PROGRAM MAIN
VAR
	bError						: BOOL;					// True if modules have errors
		(***** Axis variable *****)
	lrAxisVelo					: LREAL;
		
		(***** Variables of state machine *****)
	bStarted					: BOOL;					// True if state machine is in state EXECUTE
	bStopped					: BOOL;					// True if state machine is in state STOPPED
	bReset						AT %Q*: BOOL;			// True if state machine is in state RESETTING
	bAborted					: BOOL;					// True if state machine is in state ABORTED
	bIdle						: BOOL;					// True if state machine is in state IDLE
	bAuto						: BOOL;					// True if state machine is in mode AUTOMATIC
	bSemi						: BOOL;					// True if state machine is in mode SEMIAUTOMATIC
	bManual						: BOOL;					// True if state machine is in mode MANUAL
	bMaintenance				: BOOL;					// True if state machine is in mode MAINTENANCE
	bStartButtonOff				: BOOL;					// To turn off start button

(* ========================== Function block instances =============================== *)

		(**** Machine elements *****)
	fbSeparateModule			: FB_SeparatingModule;			// Separating module
	fbMetalSorting				: FB_SortingModule;				// Module that sorts metal boxes
	fbPlasticSorting			: FB_SortingModule;				// Module that sorts plastic boxes
	fbComprAir					: FB_SignalHandlingIntern;		// Compressed air
	fbPowerSupply				: FB_SignalHandlingIntern;		// Power supply
	fbVisu						: FB_Visu;						// Visualization

		(***** Buttons *****)
	fbButtonStart				: FB_SignalHandlingIntern;		// Button to start the machine
	fbButtonStop				: FB_SignalHandlingIntern;		// Button to stop the machine
	fbButtonReset				: FB_SignalHandlingIntern;		// Button to reset the machine
	fbButtonAbort				: FB_SignalHandlingIntern;		// Button to abort the machine
	fbButtonAuto				: FB_SignalHandlingIntern;		// Button to change machine mode to AUTOMATIC
	fbButtonSemi				: FB_SignalHandlingIntern;		// Button to change machine mode to SEMI-AUTOMATIC
	fbButtonManual				: FB_SignalHandlingIntern;		// Button to change machine mode to MANUAL
	fbButtonMaintenance			: FB_SignalHandlingIntern;		// Button to change machine mode to MAINTENANCE
	fbButtonPower				: FB_SignalHandlingIntern;		// Button to control power supply
	fbButtonComprAir			: FB_SignalHandlingIntern;		// Button to control compressed air

(* ========================== COMMON VARIABLES =============================== *)	

		(***** State machine *****)
	fbStateMachineAuto			: PS_PackML_StateMachine_Auto;			// State machine for mode AUTOMATIC
	fbStateMachineSemiAuto		: PS_PackML_StateMachine_SemiAuto;		// State machine for mode SEMI-AUTOMATIC
	fbStateMachineManual		: PS_PackML_StateMachine_Manual;		// State machine for mode MANUAL
	fbStateMachineMaintenance	: PS_PackML_StateMachine_Maintenance;	// State machine for mode MAINTENANCE
	
	ePMLUnitMode				: E_PMLUnitMode := ePMLUnitMode_IDLE;	// Current mode
	ePMLUnitModeRequested		: E_PMLUnitMode;						// Requested mode
	fbUnitModeManager			: PS_UnitModeManager;					// Mode manager
	ePMLState					: E_PMLState := ePMLState_IDLE;			// Current state
	ePMLStateRequested			: E_PMLState;							// Requested state
	
		(* Common variables *)
	bManualAxisEnable			: BOOL;							// True if it is allowed to move manually axis
	fbTriggerStart				: R_TRIG;						// To diagnose rising edge of start button
	fbTriggerSeparated			: R_TRIG;						// To diagnose rising edge of separated box
	fbTriggerSelectedM			: R_TRIG;						// To diagnose rising edge of selected metal box
	fbTriggerSelectedP			: R_TRIG;						// To diagnose rising edge of selected plastic box
	nBoxesOnTheWay				: INT;							// Number of boxes being moved
	aClampTemps					: ARRAY[1..100] OF LREAL;		// Temperature of clamp cylinder
	aBarrierTemps				: ARRAY[1..100] OF LREAL;		// Temperature of barrier cylinder
	aMetalTemps					: ARRAY[1..100] OF LREAL;		// Temperature of metal cylinder
	aPlasticTemps				: ARRAY[1..100] OF LREAL;		// Temperature of plastic cylinder
	bStartingStart				: BOOL;							// True if state machine is in state STARTING
	bResetStart					: BOOL;							// True if state machine is in state RESETTING
	bHaltStart					: BOOL;							// True if state machine is in state STOPPING
	nHaltTriesSeperate			: INT;
	nHaltTriesMetal				: INT;
	nHaltTriesPlastic			: INT;
END_VAR

// =========================================================
	// Getting errors of modules
	
bError := fbSeparateModule.fbAxis.iErrorID <> 0
			OR fbMetalSorting.fbAxis.iErrorID <> 0
			OR fbPlasticSorting.fbAxis.iErrorID <> 0
			OR fbSeparateModule.bClampError OR fbSeparateModule.bBarrierError
			OR fbMetalSorting.bCylError OR fbPlasticSorting.bCylError;
	
// =========================================================
	// Setting velocities of axes

IF ePMLUnitMode = ePMLUnitMode_AUTOMATIC OR ePMLUnitMode = ePMLUnitMode_SEMIAUTOMATIC THEN
	lrAxisVelo := 100;
ELSE
	lrAxisVelo := 50;
END_IF

// =========================================================
	// Noticing separated and selected boxes
	
fbTriggerSeparated( CLK := fbSeparateModule.bSeparated );
fbTriggerSelectedM( CLK := fbMetalSorting.bSelected );
fbTriggerSelectedP( CLK := fbPlasticSorting.bSelected );
						
// =========================================================
	// Getting cylinder temperatures of modules
	
aBarrierTemps 	:= fbSeparateModule.aBarrierTemps;
aClampTemps 	:= fbSeparateModule.aClampTemps;
aMetalTemps 	:= fbMetalSorting.aTemps;
aPlasticTemps 	:= fbPlasticSorting.aTemps;

// =========================================================
	// Cylinder options of modules
	
fbSeparateModule.M_CylinderOptions();
fbMetalSorting.M_CylinderOptions();
fbPlasticSorting.M_CylinderOptions();

// =========================================================
	// Mode and state requests
A_Requests();

	// Enable for power supply, compressed air control and buttons
A_Enable();

	// Input variables of separating and sorting modules
A_ModuleInputs();

	// Output variables
A_SetOutput();

	// State machine
A_StateMachine();

	// Visualization
A_Visu();

// =========================================================

ACTION A_Semiautomatic:
// =========================================================

CASE ePMLState OF
	
// =========================================================
	// Turning axis reset off, passing it to axis instances
	ePMLState_IDLE:		

				IF bResetStart THEN
					bResetStart 			:= FALSE;
					
					fbSeparateModule.bReset	:= FALSE;
					fbSeparateModule.M_Reset();
					
					fbMetalSorting.bReset 	:= FALSE;
					fbMetalSorting.M_Reset();
					
					fbPlasticSorting.bReset	:= FALSE;
					fbPlasticSorting.M_Reset();
					
					fbStateMachineSemiAuto.StateComplete := FALSE;
				END_IF
	
// =========================================================
	// Resetting variables for executing automatic mode, checking status of axes
	ePMLState_STARTING:	

				IF NOT bStartingStart THEN
					bStartingStart 				:= TRUE;
					
					fbSeparateModule.bStarting	:= TRUE;
					fbSeparateModule.M_Starting();
					
					fbMetalSorting.bStarting 	:= TRUE;
					fbMetalSorting.M_Starting();
					
					fbPlasticSorting.bStarting	:= TRUE;
					fbPlasticSorting.M_Starting();
				END_IF

				IF NOT fbSeparateModule.bStartingDone THEN
					fbSeparateModule.M_Starting();
				END_IF
				
				IF NOT fbMetalSorting.bStartingDone THEN
					fbMetalSorting.M_Starting();
				END_IF
				
				IF NOT fbPlasticSorting.bStartingDone THEN
					fbPlasticSorting.M_Starting();
				END_IF

				IF fbSeparateModule.bStartingDone AND fbMetalSorting.bStartingDone
				AND fbPlasticSorting.bStartingDone THEN
					fbStateMachineSemiAuto.StateComplete := TRUE;
				END_IF

// =========================================================
	// Executing semi-automatic mode
	ePMLState_EXECUTE:	

				IF bStartingStart THEN
					bStartingStart 				:= FALSE;
					
					fbSeparateModule.bStarting 	:= FALSE;
					fbSeparateModule.M_Starting();
					
					fbMetalSorting.bStarting 	:= FALSE;
					fbMetalSorting.M_Starting();
					
					fbPlasticSorting.bStarting 	:= FALSE;
					fbPlasticSorting.M_Starting();
					
					fbStateMachineSemiAuto.StateComplete := FALSE;
				END_IF
				
				fbSeparateModule.M_Semiautomatic();
				fbMetalSorting.M_Semiautomatic();
				fbPlasticSorting.M_Semiautomatic();
				
				IF fbTriggerSeparated.Q THEN
					nBoxesOnTheWay := nBoxesOnTheWay + 1;
				END_IF
				
				IF fbTriggerSelectedM.Q THEN
					nBoxesOnTheWay := nBoxesOnTheWay - 1;
				END_IF
				
				IF fbTriggerSelectedP.Q THEN
					nBoxesOnTheWay := nBoxesOnTheWay - 1;
				END_IF
						
// =========================================================
	// Stopping axes
	ePMLState_ABORTING:	

				IF NOT bHaltStart THEN
					bHaltStart 				:= TRUE;
					
					fbSeparateModule.bHalt 	:= TRUE;
					fbSeparateModule.M_Stop();
					
					fbMetalSorting.bHalt 	:= TRUE;
					fbMetalSorting.M_Stop();
					
					fbPlasticSorting.bHalt 	:= TRUE;
					fbPlasticSorting.M_Stop();						
				END_IF

				IF NOT fbSeparateModule.bHaltDone THEN
					fbSeparateModule.M_Stop();
				END_IF
				
				IF NOT fbMetalSorting.bHaltDone THEN
					fbMetalSorting.M_Stop();
				END_IF
				
				IF NOT fbPlasticSorting.bHaltDone THEN
					fbPlasticSorting.M_Stop();
				END_IF

				IF fbSeparateModule.bHaltDone AND fbMetalSorting.bHaltDone
				AND fbPlasticSorting.bHaltDone THEN
					fbStateMachineSemiAuto.StateComplete := TRUE;
				END_IF
	
// =========================================================
	// Turning off axis stop, passing it to axis instances
	ePMLState_ABORTED:	

				IF fbStateMachineSemiAuto.StateComplete THEN
					fbStateMachineSemiAuto.StateComplete := FALSE;
				END_IF
				
				IF bHaltStart THEN
					bHaltStart 				:= FALSE;
					
					fbSeparateModule.bHalt 	:= FALSE;
					fbSeparateModule.M_Stop();
					
					fbMetalSorting.bHalt 	:= FALSE;
					fbMetalSorting.M_Stop();
					
					fbPlasticSorting.bHalt 	:= FALSE;
					fbPlasticSorting.M_Stop();
				END_IF
	
// =========================================================
	ePMLState_CLEARING:	

				fbStateMachineSemiAuto.StateComplete := TRUE;
	
// =========================================================
	// Selecting boxes on conveyor belt to destination, then stopping axes
	ePMLState_STOPPING:	

				IF fbTriggerSeparated.Q THEN
					nBoxesOnTheWay := nBoxesOnTheWay + 1;
				END_IF
				
				IF fbTriggerSelectedM.Q THEN
					nBoxesOnTheWay := nBoxesOnTheWay - 1;
				END_IF
				
				IF fbTriggerSelectedP.Q THEN
					nBoxesOnTheWay := nBoxesOnTheWay - 1;
				END_IF
				
				IF nBoxesOnTheWay = 0 AND NOT bHaltStart THEN
					bHaltStart				:= TRUE;
					
					fbSeparateModule.bHalt 	:= TRUE;
					fbSeparateModule.M_Stop();
					
					fbMetalSorting.bHalt 	:= TRUE;
					fbMetalSorting.M_Stop();
					
					fbPlasticSorting.bHalt 	:= TRUE;
					fbPlasticSorting.M_Stop();						
				END_IF
				
				IF NOT fbSeparateModule.bHaltDone OR nBoxesOnTheWay <> 0 THEN
					fbSeparateModule.M_Automatic();
				END_IF
				
				IF NOT fbMetalSorting.bHaltDone OR nBoxesOnTheWay <> 0 THEN
					fbMetalSorting.M_Automatic();
				END_IF
				
				IF NOT fbPlasticSorting.bHaltDone OR nBoxesOnTheWay <> 0 THEN
					fbPlasticSorting.M_Automatic();
				END_IF

				IF fbSeparateModule.bHaltDone AND fbMetalSorting.bHaltDone
				AND fbPlasticSorting.bHaltDone AND nBoxesOnTheWay = 0 THEN
					fbStateMachineSemiAuto.StateComplete := TRUE;
				END_IF
					
// =========================================================
	// Turning off axis stop, passing it to axis instances
	ePMLState_STOPPED:	

				IF fbStateMachineSemiAuto.StateComplete THEN
					fbStateMachineSemiAuto.StateComplete := FALSE;
				END_IF
				
				IF bHaltStart THEN
					bHaltStart 				:= FALSE;
					
					fbSeparateModule.bHalt 	:= FALSE;
					fbSeparateModule.M_Stop();
					
					fbMetalSorting.bHalt 	:= FALSE;
					fbMetalSorting.M_Stop();
					
					fbPlasticSorting.bHalt 	:= FALSE;
					fbPlasticSorting.M_Stop();
				END_IF

// =========================================================
	// Resetting cylinders and axes
	ePMLState_RESETTING:	

				IF NOT bResetStart THEN
					bResetStart				:= TRUE;
					
					fbSeparateModule.bReset	:= TRUE;
					fbSeparateModule.M_Reset();
					
					fbMetalSorting.bReset 	:= TRUE;
					fbMetalSorting.M_Reset();
					
					fbPlasticSorting.bReset	:= TRUE;
					fbPlasticSorting.M_Reset();
				END_IF
				
				IF NOT fbSeparateModule.bResetDone THEN
					fbSeparateModule.M_Reset();
				END_IF
				
				IF NOT fbMetalSorting.bResetDone THEN
					fbMetalSorting.M_Reset();
				END_IF
				
				IF NOT fbPlasticSorting.bResetDone THEN
					fbPlasticSorting.M_Reset();
				END_IF
				
				IF fbSeparateModule.bResetDone AND fbMetalSorting.bResetDone AND fbPlasticSorting.bResetDone 
				AND fbSeparateModule.bClampAtBase AND fbSeparateModule.bBarrierAtBase
				AND fbMetalSorting.bAtBase AND fbPlasticSorting.bAtBase THEN
					nBoxesOnTheWay 							:= 0;
					fbStateMachineSemiAuto.StateComplete 	:= TRUE;
				END_IF
END_CASE

// =========================================================
END_ACTION

ACTION A_Maintenance:
// =========================================================

CASE ePMLState OF
	
// =========================================================
	// Turning axis reset off, passing it to axis instances
	ePMLState_IDLE:		

				IF bResetStart THEN
					bResetStart 			:= FALSE;
					
					fbSeparateModule.bReset	:= FALSE;
					fbSeparateModule.M_Reset();
					
					fbMetalSorting.bReset 	:= FALSE;
					fbMetalSorting.M_Reset();
					
					fbPlasticSorting.bReset 	:= FALSE;
					fbPlasticSorting.M_Reset();
					
					fbStateMachineMaintenance.StateComplete := FALSE;
				END_IF
	
// =========================================================
	// Checking status of axes
	ePMLState_STARTING:	

				IF NOT bStartingStart THEN
					bStartingStart 				:= TRUE;
					
					fbSeparateModule.bStarting 	:= TRUE;
					fbSeparateModule.M_Starting();
					
					fbMetalSorting.bStarting 	:= TRUE;
					fbMetalSorting.M_Starting();
					
					fbPlasticSorting.bStarting 	:= TRUE;
					fbPlasticSorting.M_Starting();
				END_IF

				IF NOT fbSeparateModule.bStartingDone THEN
					fbSeparateModule.M_Starting();
				END_IF
				
				IF NOT fbMetalSorting.bStartingDone THEN
					fbMetalSorting.M_Starting();
				END_IF
				
				IF NOT fbPlasticSorting.bStartingDone THEN
					fbPlasticSorting.M_Starting();
				END_IF

				IF fbSeparateModule.bStartingDone AND fbMetalSorting.bStartingDone
				AND fbPlasticSorting.bStartingDone THEN
					fbStateMachineMaintenance.StateComplete := TRUE;
				END_IF

// =========================================================
	// Executing maintenance mode
	ePMLState_EXECUTE:	

				IF bStartingStart THEN
					bStartingStart 				:= FALSE;
					
					fbSeparateModule.bStarting 	:= FALSE;
					fbSeparateModule.M_Starting();
					
					fbMetalSorting.bStarting 	:= FALSE;
					fbMetalSorting.M_Starting();
					
					fbPlasticSorting.bStarting 	:= FALSE;
					fbPlasticSorting.M_Starting();
					
					fbStateMachineMaintenance.StateComplete := FALSE;
				END_IF
				
				fbSeparateModule.M_Maintenance();
				fbMetalSorting.M_Maintenance();
				fbPlasticSorting.M_Maintenance();
						
// =========================================================
	// Stopping axes
	ePMLState_ABORTING:	

				IF NOT bHaltStart THEN
					bHaltStart 				:= TRUE;
					
					fbSeparateModule.bHalt 	:= TRUE;
					fbSeparateModule.M_Stop();
					
					fbMetalSorting.bHalt 	:= TRUE;
					fbMetalSorting.M_Stop();
					
					fbPlasticSorting.bHalt 	:= TRUE;
					fbPlasticSorting.M_Stop();						
				END_IF

				IF NOT fbSeparateModule.bHaltDone THEN
					fbSeparateModule.M_Stop();
				END_IF
				
				IF NOT fbMetalSorting.bHaltDone THEN
					fbMetalSorting.M_Stop();
				END_IF
				
				IF NOT fbPlasticSorting.bHaltDone THEN
					fbPlasticSorting.M_Stop();
				END_IF

				IF fbSeparateModule.bHaltDone AND fbMetalSorting.bHaltDone
				AND fbPlasticSorting.bHaltDone THEN
					fbStateMachineMaintenance.StateComplete := TRUE;
				END_IF
	
// =========================================================
	// Turning off axis stop, passing it to axis instances
	ePMLState_ABORTED:	

				IF fbStateMachineMaintenance.StateComplete THEN
					fbStateMachineMaintenance.StateComplete := FALSE;
				END_IF
				
				IF bHaltStart THEN
					bHaltStart 				:= FALSE;
					
					fbSeparateModule.bHalt 	:= FALSE;
					fbSeparateModule.M_Stop();
					
					fbMetalSorting.bHalt 	:= FALSE;
					fbMetalSorting.M_Stop();
					
					fbPlasticSorting.bHalt 	:= FALSE;
					fbPlasticSorting.M_Stop();
				END_IF
	
// =========================================================
	ePMLState_CLEARING:	

				fbStateMachineMaintenance.StateComplete := TRUE;
	
// =========================================================
	// Stopping axes
	ePMLState_STOPPING:	

				IF NOT bHaltStart THEN
					bHaltStart 				:= TRUE;
					
					fbSeparateModule.bHalt 	:= TRUE;
					fbSeparateModule.M_Stop();
					
					fbMetalSorting.bHalt 	:= TRUE;
					fbMetalSorting.M_Stop();
					
					fbPlasticSorting.bHalt 	:= TRUE;
					fbPlasticSorting.M_Stop();					
				END_IF

				IF NOT fbSeparateModule.bHaltDone THEN
					fbSeparateModule.M_Stop();
				END_IF
				
				IF NOT fbMetalSorting.bHaltDone THEN
					fbMetalSorting.M_Stop();
				END_IF
				
				IF NOT fbPlasticSorting.bHaltDone THEN
					fbPlasticSorting.M_Stop();
				END_IF

				IF fbSeparateModule.bHaltDone AND fbMetalSorting.bHaltDone
					AND fbPlasticSorting.bHaltDone THEN
						fbStateMachineMaintenance.StateComplete := TRUE;
				END_IF
					
// =========================================================
	// Turning off axis stop, passing it to axis instances
	ePMLState_STOPPED:	

				IF fbStateMachineMaintenance.StateComplete THEN
					fbStateMachineMaintenance.StateComplete := FALSE;
				END_IF
				
				IF bHaltStart THEN
					bHaltStart 				:= FALSE;
					
					fbSeparateModule.bHalt 	:= FALSE;
					fbSeparateModule.M_Stop();
					
					fbMetalSorting.bHalt 	:= FALSE;
					fbMetalSorting.M_Stop();
					
					fbPlasticSorting.bHalt 	:= FALSE;
					fbPlasticSorting.M_Stop();
				END_IF

// =========================================================
	// Resetting cylinders and axes
	ePMLState_RESETTING:	

				IF NOT bResetStart THEN
					bResetStart 			:= TRUE;
					
					fbSeparateModule.bReset	:= TRUE;
					fbSeparateModule.M_Reset();
					
					fbMetalSorting.bReset 	:= TRUE;
					fbMetalSorting.M_Reset();
					
					fbPlasticSorting.bReset	:= TRUE;
					fbPlasticSorting.M_Reset();
				END_IF
				
				IF NOT fbSeparateModule.bResetDone THEN
					fbSeparateModule.M_Reset();
				END_IF
				
				IF NOT fbMetalSorting.bResetDone THEN
					fbMetalSorting.M_Reset();
				END_IF
				
				IF NOT fbPlasticSorting.bResetDone THEN
					fbPlasticSorting.M_Reset();
				END_IF
				
				IF fbSeparateModule.bResetDone AND fbMetalSorting.bResetDone AND fbPlasticSorting.bResetDone 
				AND fbSeparateModule.bClampAtBase AND fbSeparateModule.bBarrierAtBase
				AND fbMetalSorting.bAtBase AND fbPlasticSorting.bAtBase THEN
					fbStateMachineMaintenance.StateComplete := TRUE;
				END_IF
END_CASE

// =========================================================
END_ACTION

ACTION A_SetOutput:
// =========================================================
		// State variables

bStopped 		:= (ePMLState = ePMLState_STOPPED);
bStarted 		:= (ePMLState = ePMLState_EXECUTE);
bReset 			:= (ePMLState = ePMLState_RESETTING);
bAborted 		:= (ePMLState = ePMLState_ABORTED);
bIdle 			:= (ePMLState = ePMLState_IDLE AND fbPowerSupply.bOut);

// =========================================================
		// Mode variables

bAuto 			:= (ePMLUnitMode = ePMLUnitMode_AUTOMATIC);
bSemi 			:= (ePMLUnitMode = ePMLUnitMode_SEMIAUTOMATIC);
bManual 		:= (ePMLUnitMode = ePMLUnitMode_MANUAL);
bMaintenance 	:= (ePMLUnitMode = ePMLUnitMode_MAINTENANCE);

// =========================================================
		// Power supply and compressed air control
		
fbPowerSupply.M_SetOutput();
fbComprAir.M_SetOutput();		

// =========================================================
		// Modules

fbSeparateModule.M_SetOutput();
fbMetalSorting.M_SetOutput();
fbPlasticSorting.M_SetOutput();

// =========================================================
		// Buttons

	// Power supply and compressed air control
fbButtonPower.M_SetOutput();
fbButtonComprAir.M_SetOutput();	

	// States
fbButtonStart.M_SetOutput();
fbButtonStop.M_SetOutput();
fbButtonReset.M_SetOutput();
fbButtonAbort.M_SetOutput();

	// Modes
fbButtonAuto.M_SetOutput();
fbButtonSemi.M_SetOutput();
fbButtonManual.M_SetOutput();
fbButtonMaintenance.M_SetOutput();	
	
// =========================================================
END_ACTION

ACTION A_Requests:
// =========================================================
	// Check for state requests

fbTriggerStart( CLK := fbButtonStart.bOut);

IF bStartButtonOff AND NOT fbButtonStart.bInput THEN
	bStartButtonOff := FALSE;
END_IF

IF fbTriggerStart.Q THEN
	bStartButtonOff := TRUE;

	IF ePMLState = ePMLState_ABORTED THEN
		ePMLStateRequested := ePMLState_CLEARING;
		
	ELSIF ePMLState = ePMLState_STOPPED THEN
		ePMLStateRequested := ePMLState_RESETTING;
		
	ELSIF ePMLState = ePMLState_IDLE AND fbPowerSupply.bOut THEN
		ePMLStateRequested := ePMLState_STARTING;
	END_IF
	
ELSIF fbButtonStop.bOut THEN
	ePMLStateRequested := ePMLState_STOPPING;
	
ELSIF fbButtonReset.bOut THEN
	ePMLStateRequested := ePMLState_RESETTING;
END_IF

// =========================================================
	// Check for mode requests

IF fbButtonManual.bOut THEN
	ePMLUnitModeRequested := ePMLUnitMode_MANUAL;
	
ELSIF fbButtonAuto.bOut THEN
	ePMLUnitModeRequested := ePMLUnitMode_AUTOMATIC;
	
ELSIF fbButtonSemi.bOut THEN
	ePMLUnitModeRequested := ePMLUnitMode_SEMIAUTOMATIC;
	
ELSIF fbButtonMaintenance.bOut THEN
	ePMLUnitModeRequested := ePMLUnitMode_MAINTENANCE;
END_IF

IF fbButtonManual.bOut OR fbButtonAuto.bOut OR fbButtonSemi.bOut OR fbButtonMaintenance.bOut THEN
	fbUnitModeManager(	Execute 		:= TRUE,
						eModeCommand 	:= ePMLUnitModeRequested,
						ePMLState 		:= ePMLState);
END_IF

IF fbUnitModeManager.Done THEN
	ePMLUnitMode := fbUnitModeManager.eModeStatus;
	
	fbUnitModeManager(Execute := FALSE);
END_IF
// =========================================================
END_ACTION

ACTION A_Manual:
// =========================================================

CASE ePMLState OF
	
// =========================================================
	// Turning axis reset off, passing it to axis instances
	ePMLState_IDLE:		

				IF bResetStart THEN
					bResetStart 			:= FALSE;
					
					fbSeparateModule.bReset	:= FALSE;
					fbSeparateModule.M_Reset();
					
					fbMetalSorting.bReset 	:= FALSE;
					fbMetalSorting.M_Reset();
					
					fbPlasticSorting.bReset	:= FALSE;
					fbPlasticSorting.M_Reset();
					
					fbStateMachineManual.StateComplete := FALSE;
				END_IF
	
// =========================================================
	// Checking status of axes
	ePMLState_STARTING:	

				IF NOT bStartingStart THEN
					bStartingStart 				:= TRUE;
					
					fbSeparateModule.bStarting 	:= TRUE;
					fbSeparateModule.M_Starting();
					
					fbMetalSorting.bStarting 	:= TRUE;
					fbMetalSorting.M_Starting();
					
					fbPlasticSorting.bStarting 	:= TRUE;
					fbPlasticSorting.M_Starting();
				END_IF

				IF NOT fbSeparateModule.bStartingDone THEN
					fbSeparateModule.M_Starting();
				END_IF
				
				IF NOT fbMetalSorting.bStartingDone THEN
					fbMetalSorting.M_Starting();
				END_IF
				
				IF NOT fbPlasticSorting.bStartingDone THEN
					fbPlasticSorting.M_Starting();
				END_IF

				IF fbSeparateModule.bStartingDone AND fbMetalSorting.bStartingDone
				AND fbPlasticSorting.bStartingDone THEN
					fbStateMachineManual.StateComplete := TRUE;
				END_IF

// =========================================================
	// Executing manual mode
	ePMLState_EXECUTE:	

				IF bStartingStart THEN
					bStartingStart 				:= FALSE;
					
					fbSeparateModule.bStarting 	:= FALSE;
					fbSeparateModule.M_Starting();
					
					fbMetalSorting.bStarting 	:= FALSE;
					fbMetalSorting.M_Starting();
					
					fbPlasticSorting.bStarting 	:= FALSE;
					fbPlasticSorting.M_Starting();
					
					fbStateMachineManual.StateComplete := FALSE;
				END_IF
				
				fbSeparateModule.M_Manual();
				fbMetalSorting.M_Manual();
				fbPlasticSorting.M_Manual();
						
// =========================================================
	// Stopping axes
	ePMLState_ABORTING:	

				IF NOT bHaltStart THEN
					bHaltStart 				:= TRUE;
					
					fbSeparateModule.bHalt 	:= TRUE;
					fbSeparateModule.M_Stop();
					
					fbMetalSorting.bHalt 	:= TRUE;
					fbMetalSorting.M_Stop();
					
					fbPlasticSorting.bHalt 	:= TRUE;
					fbPlasticSorting.M_Stop();						
				END_IF

				IF NOT fbSeparateModule.bHaltDone THEN
					fbSeparateModule.M_Stop();
				END_IF
				
				IF NOT fbMetalSorting.bHaltDone THEN
					fbMetalSorting.M_Stop();
				END_IF
				
				IF NOT fbPlasticSorting.bHaltDone THEN
					fbPlasticSorting.M_Stop();
				END_IF

				IF fbSeparateModule.bHaltDone AND fbMetalSorting.bHaltDone
				AND fbPlasticSorting.bHaltDone THEN
					fbStateMachineManual.StateComplete := TRUE;
				END_IF
	
// =========================================================
	// Turning off axis stop, passing it to axis instances
	ePMLState_ABORTED:	

				IF fbStateMachineManual.StateComplete THEN
					fbStateMachineManual.StateComplete := FALSE;
				END_IF
				
				IF bHaltStart THEN
					bHaltStart 				:= FALSE;
					
					fbSeparateModule.bHalt 	:= FALSE;
					fbSeparateModule.M_Stop();
					
					fbMetalSorting.bHalt 	:= FALSE;
					fbMetalSorting.M_Stop();
					
					fbPlasticSorting.bHalt 	:= FALSE;
					fbPlasticSorting.M_Stop();
				END_IF
	
// =========================================================
	ePMLState_CLEARING:	

				fbStateMachineManual.StateComplete := TRUE;
	
// =========================================================
	// Stopping axes
	ePMLState_STOPPING:	

				IF NOT bHaltStart THEN
					bHaltStart 				:= TRUE;
					
					fbSeparateModule.bHalt 	:= TRUE;
					fbSeparateModule.M_Stop();
					
					fbMetalSorting.bHalt 	:= TRUE;
					fbMetalSorting.M_Stop();
					
					fbPlasticSorting.bHalt 	:= TRUE;
					fbPlasticSorting.M_Stop();					
				END_IF

				IF NOT fbSeparateModule.bHaltDone THEN
					fbSeparateModule.M_Stop();
				END_IF
				
				IF NOT fbMetalSorting.bHaltDone THEN
					fbMetalSorting.M_Stop();
				END_IF
				
				IF NOT fbPlasticSorting.bHaltDone THEN
					fbPlasticSorting.M_Stop();
				END_IF

				IF fbSeparateModule.bHaltDone AND fbMetalSorting.bHaltDone
				AND fbPlasticSorting.bHaltDone THEN
					fbStateMachineManual.StateComplete := TRUE;
				END_IF
					
// =========================================================
	// Turning off axis stop, passing it to axis instances
	ePMLState_STOPPED:	

				IF fbStateMachineManual.StateComplete THEN
					fbStateMachineManual.StateComplete := FALSE;
				END_IF
				
				IF bHaltStart THEN
					bHaltStart 				:= FALSE;
					
					fbSeparateModule.bHalt 	:= FALSE;
					fbSeparateModule.M_Stop();
					
					fbMetalSorting.bHalt 	:= FALSE;
					fbMetalSorting.M_Stop();
					
					fbPlasticSorting.bHalt 	:= FALSE;
					fbPlasticSorting.M_Stop();
				END_IF

// =========================================================
	// Resetting cylinders and axes
	ePMLState_RESETTING:	

				IF NOT bResetStart THEN
					bResetStart 			:= TRUE;
					
					fbSeparateModule.bReset	:= TRUE;
					fbSeparateModule.M_Reset();
					
					fbMetalSorting.bReset 	:= TRUE;
					fbMetalSorting.M_Reset();
					
					fbPlasticSorting.bReset	:= TRUE;
					fbPlasticSorting.M_Reset();
				END_IF
				
				IF NOT fbSeparateModule.bResetDone THEN
					fbSeparateModule.M_Reset();
				END_IF
				
				IF NOT fbMetalSorting.bResetDone THEN
					fbMetalSorting.M_Reset();
				END_IF
				
				IF NOT fbPlasticSorting.bResetDone THEN
					fbPlasticSorting.M_Reset();
				END_IF
				
				IF fbSeparateModule.bResetDone AND fbMetalSorting.bResetDone AND fbPlasticSorting.bResetDone 
				AND fbSeparateModule.bClampAtBase AND fbSeparateModule.bBarrierAtBase
				AND fbMetalSorting.bAtBase AND fbPlasticSorting.bAtBase THEN
					fbStateMachineManual.StateComplete := TRUE;
				END_IF
END_CASE

// =========================================================
END_ACTION

ACTION A_Enable:
// =========================================================
		// Power supply

fbButtonPower.bEnable 	:= TRUE;
fbPowerSupply.bInput 	:= fbButtonPower.bOut;
fbPowerSupply.bEnable 	:= TRUE;

// =========================================================
		// Enable of axes

IF ePMLState = ePMLState_ABORTED THEN
	fbSeparateModule.bAxisEnable 	:= FALSE;
	fbMetalSorting.bAxisEnable 		:= FALSE;
	fbPlasticSorting.bAxisEnable 	:= FALSE;
	
ELSIF fbPowerSupply.bOut THEN
	fbSeparateModule.bAxisEnable 	:= TRUE;
	fbMetalSorting.bAxisEnable 		:= TRUE;
	fbPlasticSorting.bAxisEnable 	:= TRUE;
END_IF

// =========================================================
		// Manual axis control
		
bManualAxisEnable := fbPowerSupply.bOut AND (ePMLState = ePMLState_EXECUTE)
					AND ((ePMLUnitMode = ePMLUnitMode_MANUAL) OR (ePMLUnitMode = ePMLUnitMode_MAINTENANCE));
					
fbSeparateModule.bManualAxisEnable 	:= bManualAxisEnable;
fbMetalSorting.bManualAxisEnable 	:= bManualAxisEnable;
fbPlasticSorting.bManualAxisEnable 	:= bManualAxisEnable;

// =========================================================
		// Compressed air control
	
IF ePMLUnitMode <> ePMLUnitMode_MAINTENANCE THEN
	fbComprAir.bInput := fbPowerSupply.bOut;
ELSE
	fbComprAir.bInput := fbButtonComprAir.bOut;
END_IF

fbComprAir.bEnable 			:= TRUE;
fbButtonComprAir.bEnable 	:= ePMLUnitMode = ePMLUnitMode_MAINTENANCE;

// =========================================================
		// Enable of sensors
		
fbSeparateModule.bSensorEnable 	:= TRUE;
fbMetalSorting.bSensorEnable 	:= TRUE;
fbPlasticSorting.bSensorEnable 	:= TRUE;

// =========================================================
		// Enable actions of modules

fbSeparateModule.M_Enable();
fbMetalSorting.M_Enable();
fbPlasticSorting.M_Enable();

// =========================================================
		// States and modes
		
	// Start button
fbButtonStart.bEnable	 := NOT (ePMLState = ePMLState_IDLE AND bError);
	// Stop button
fbButtonStop.bEnable 	:= ePMLState = ePMLState_STOPPING OR ePMLState = ePMLState_EXECUTE OR ePMLState = ePMLState_IDLE;
	// Reset button
fbButtonReset.bEnable	:= (ePMLState = ePMLState_STOPPED);
	// Abort button
fbButtonAbort.bInput 	:= NOT fbPowerSupply.bOut;
fbButtonAbort.bEnable 	:= (ePMLState = ePMLState_EXECUTE OR ePMLState = ePMLState_STOPPING
							OR ePMLState = ePMLState_RESETTING);
	// Automatic mode button
fbButtonAuto.bEnable 		:= ePMLUnitMode <> ePMLUnitMode_AUTOMATIC AND ePMLState = ePMLState_IDLE;
	// Semi-automatic mode button *)
fbButtonSemi.bEnable 		:= ePMLUnitMode <> ePMLUnitMode_SEMIAUTOMATIC AND ePMLState = ePMLState_IDLE;
	// Manual mode button
fbButtonManual.bEnable 		:= ePMLUnitMode <> ePMLUnitMode_MANUAL AND ePMLState = ePMLState_IDLE;
	// Maintenance mode button
fbButtonMaintenance.bEnable	:= ePMLUnitMode <> ePMLUnitMode_MAINTENANCE AND ePMLState = ePMLState_IDLE;

// =========================================================
END_ACTION

ACTION A_StateMachine:
// =========================================================
	// Mode and state handling
	
CASE ePMLUnitMode OF
	
	ePMLUnitMode_AUTOMATIC:		

				fbStateMachineAuto(	Start 	:= ePMLStateRequested = ePMLState_STARTING,
									Stop 	:= fbButtonStop.bOut,
									Reset 	:= fbButtonReset.bOut OR ePMLStateRequested = ePMLState_RESETTING,
									Clear 	:= ePMLStateRequested = ePMLState_CLEARING,
									Abort 	:= fbButtonAbort.bOut OR (bError AND ePMLState = ePMLState_EXECUTE));
								 
				ePMLState := fbStateMachineAuto.ePMLState;
				
				A_Automatic();

// =========================================================	
	ePMLUnitMode_MANUAL:		

				fbStateMachineManual(	Start 	:= ePMLStateRequested = ePMLState_STARTING,
										Stop 	:= fbButtonStop.bOut,
										Reset 	:= fbButtonReset.bOut OR ePMLStateRequested = ePMLState_RESETTING,
										Clear 	:= ePMLStateRequested = ePMLState_CLEARING,
										Abort 	:= fbButtonAbort.bOut OR (bError AND ePMLState = ePMLState_EXECUTE));
									 
				ePMLState := fbStateMachineManual.ePMLState;
				
				A_Manual();
	
// =========================================================						
	ePMLUnitMode_SEMIAUTOMATIC:	

				fbStateMachineSemiAuto(	Start 	:= ePMLStateRequested = ePMLState_STARTING,
									 	Stop 	:= fbButtonStop.bOut,
										Reset 	:= fbButtonReset.bOut OR ePMLStateRequested = ePMLState_RESETTING,
										Clear 	:= ePMLStateRequested = ePMLState_CLEARING,
										Abort 	:= fbButtonAbort.bOut OR (bError AND ePMLState = ePMLState_EXECUTE));
									 
				ePMLState := fbStateMachineSemiAuto.ePMLState;
				
				A_Semiautomatic();
	
// =========================================================						
	ePMLUnitMode_MAINTENANCE:	

				fbStateMachineMaintenance(	Start 	:= ePMLStateRequested = ePMLState_STARTING,
											Stop 	:= fbButtonStop.bOut,
											Reset 	:= fbButtonReset.bOut OR ePMLStateRequested = ePMLState_RESETTING,
											Clear 	:= ePMLStateRequested = ePMLState_CLEARING,
											Abort 	:= fbButtonAbort.bOut OR (bError AND ePMLState = ePMLState_EXECUTE));
									 
				ePMLState := fbStateMachineMaintenance.ePMLState;
				
				A_Maintenance();
END_CASE

// =========================================================
END_ACTION

ACTION A_Visu:
// =========================================================
		// Calling visu function block
		
fbVisu(	bError  				:= bError, 
		lrAxisVelo 				:= lrAxisVelo, 
		bComprAirEnabled 		:= fbComprAir.bOut, 
		bPowerEnabled 			:= fbPowerSupply.bOut, 
		bMainAxisMoves 			:= fbSeparateModule.bAxisMoves, 
		bMetalAxisMoves 		:= fbMetalSorting.bAxisMoves, 
		bPlasticAxisMoves 		:= fbPlasticSorting.bAxisMoves, 
		bClampToWork 			:= fbSeparateModule.bClampToWork, 
		bBarrierToWork 			:= fbSeparateModule.bBarrierToWork, 
		bMetalToWork 			:= fbMetalSorting.bToWork, 
		bPlasticToWork 			:= fbPlasticSorting.bToWork, 
		bClampError 			:= fbSeparateModule.bClampError, 
		sClampErrMsg 			:= fbSeparateModule.sClampErrorMsg, 
		bMetalCylError 			:= fbMetalSorting.bCylError, 
		sMetalErrMsg 			:= fbMetalSorting.sCylErrorMsg, 
		bPlasticCylError 		:= fbPlasticSorting.bCylError, 
		sPlasticErrMsg 			:= fbPlasticSorting.sCylErrorMsg, 
		nMainAxisErrorId 		:= fbSeparateModule.fbAxis.iErrorID, 
		nMetalAxisErrorId 		:= fbMetalSorting.fbAxis.iErrorID, 
		nPlasticAxisErrorId		:= fbPlasticSorting.fbAxis.iErrorID, 
		bStarted 				:= bStarted, 
		bStopped 				:= bStopped, 
		bReset 					:= bReset, 
		bAborted 				:= bAborted, 
		bIdle					:= bIdle, 
		bAuto 					:= bAuto, 
		bSemi 					:= bSemi, 
		bManual 				:= bManual, 
		bMaintenance 			:= bMaintenance, 
		bStartButtonOff 		:= bStartButtonOff, 
		bButtonPowerIn 			:= fbButtonPower.bOut, 
		bButtonComprAirIn 		:= fbButtonComprAir.bOut, 
		bButtonStartIn 			:= fbButtonStart.bOut, 
		bButtonStopIn 			:= fbButtonStop.bOut, 
		bButtonResetIn 			:= fbButtonReset.bOut, 
		bButtonAbortIn 			:= fbButtonAbort.bOut, 
		bButtonAutoIn 			:= fbButtonAuto.bOut, 
		bButtonSemiIn 			:= fbButtonSemi.bOut, 
		bButtonManuIn 			:= fbButtonManual.bOut, 
		bButtonMaintenanceIn 	:= fbButtonMaintenance.bOut, 
		bButtonMainFwIn 		:= fbSeparateModule.bButtonAxisFwOut,
		bButtonMainBwIn 		:= fbSeparateModule.bButtonAxisBwOut, 
		bButtonMetalFwIn 		:= fbMetalSorting.bButtonAxisFwOut, 
		bButtonMetalBwIn 		:= fbMetalSorting.bButtonAxisBwOut, 
		bButtonPlasticFwIn 		:= fbPlasticSorting.bButtonAxisFwOut, 
		bButtonPlasticBwIn 		:= fbPlasticSorting.bButtonAxisBwOut, 
		bButtonClampToWorkIn 	:= fbSeparateModule.bButtonClampToWorkOut, 
		bButtonBarrierToWorkIn 	:= fbSeparateModule.bButtonBarrierToWorkOut, 
		bButtonMetalToWorkIn 	:= fbMetalSorting.bButtonCylToWorkOut, 
		bButtonPlasticToWorkIn 	:= fbPlasticSorting.bButtonCylToWorkOut, 
		
		bButtonPowerOut			=> fbButtonPower.bInput, 
		bButtonComprAirOut 		=> fbButtonComprAir.bInput, 
		bButtonStartOut 		=> fbButtonStart.bInput, 
		bButtonStopOut 			=> fbButtonStop.bInput, 
		bButtonResetOut 		=> fbButtonReset.bInput, 
		bButtonAutoOut 			=> fbButtonAuto.bInput, 
		bButtonSemiOut 			=> fbButtonSemi.bInput, 
		bButtonManuOut 			=> fbButtonManual.bInput, 
		bButtonMaintenanceOut 	=> fbButtonMaintenance.bInput, 
		bButtonMainFwOut 		=> fbSeparateModule.bButtonAxisFwIn, 
		bButtonMainBwOut 		=> fbSeparateModule.bButtonAxisBwIn, 
		bButtonMetalFwOut 		=> fbMetalSorting.bButtonAxisFwIn, 
		bButtonMetalBwOut 		=> fbMetalSorting.bButtonAxisBwIn, 
		bButtonPlasticFwOut		=> fbPlasticSorting.bButtonAxisFwIn, 
		bButtonPlasticBwOut		=> fbPlasticSorting.bButtonAxisBwIn, 
		bButtonClampToWorkOut 	=> fbSeparateModule.bButtonClampToWorkIn, 
		bButtonBarrierToWorkOut	=> fbSeparateModule.bButtonBarrierToWorkIn, 
		bButtonMetalToWorkOut 	=> fbMetalSorting.bButtonCylToWorkIn, 
		bButtonPlasticToWorkOut	=> fbPlasticSorting.bButtonCylToWorkIn);
	
// =========================================================
END_ACTION

ACTION A_ModuleInputs:
// =========================================================
		// Separating modul

	// Compressed air, state and button signals
fbSeparateModule.bComprAirEnabled 	:= fbComprAir.bOut;
fbSeparateModule.bExecute 			:= ePMLState = ePMLState_EXECUTE;
fbSeparateModule.bSemiStart 		:= fbTriggerStart.Q;

	// Choose desired clamp cylinder
fbSeparateModule.bClampDiag 	:= TRUE;
fbSeparateModule.bClampTemp 	:= TRUE;
fbSeparateModule.bClampRecord 	:= FALSE;

	// Choose desired barrier cylinder
fbSeparateModule.bBarrierDiag 	:= FALSE;
fbSeparateModule.bBarrierTemp 	:= TRUE;
fbSeparateModule.bBarrierRecord	:= TRUE;

	// Axis velocity
fbSeparateModule.lrAxisVelo 	:= lrAxisVelo;

	// Timer values for clamp cylinder
fbSeparateModule.tTimeOutClamp 			:= T#2.5S;
fbSeparateModule.tRecordIntervallClamp	:= T#1S;

	// Timer values for barrier cylinder
fbSeparateModule.tTimeOutBarrier 			:= T#3S;
fbSeparateModule.tRecordIntervallBarrier 	:= T#1S;

	// Timer value for separating process
fbSeparateModule.tBarrierAtWork := T#4.5S;

	// Information about number of boxes being sorted
fbSeparateModule.iBoxesOnTheWay := nBoxesOnTheWay;

// =========================================================
		// Sorting modul for metal boxes

	// Compressed air signal
fbMetalSorting.bComprAirEnabled := fbComprAir.bOut;
	
	// Choose desired cylinder
fbMetalSorting.bCylinderDiag 	:= TRUE;
fbMetalSorting.bCylinderTemp 	:= FALSE;
fbMetalSorting.bCylinderRecord 	:= FALSE;

	// Axis velocity
fbMetalSorting.lrAxisVelo := lrAxisVelo;

	// Timer values
fbMetalSorting.tTimeOutCylinder 	:= T#3S;
fbMetalSorting.tRecordIntervall 	:= T#1S;
fbMetalSorting.tMoveAxis 			:= T#2.5S;
fbMetalSorting.tSensorDelay 		:= T#3S;

// =========================================================
		// Sorting modul for plastic boxes

	// Compressed air signal
fbPlasticSorting.bComprAirEnabled := fbComprAir.bOut;
	
	// Choose desired cylinder
fbPlasticSorting.bCylinderDiag 		:= TRUE;
fbPlasticSorting.bCylinderTemp 		:= FALSE;
fbPlasticSorting.bCylinderRecord 	:= FALSE;

	// Axis velocity
fbPlasticSorting.lrAxisVelo := lrAxisVelo;

	// Timer values
fbPlasticSorting.tTimeOutCylinder 	:= T#3S;
fbPlasticSorting.tRecordIntervall 	:= T#1S;
fbPlasticSorting.tMoveAxis 			:= T#2.5S;
fbPlasticSorting.tSensorDelay 		:= T#3S;

// =========================================================
END_ACTION

ACTION A_Automatic:
// =========================================================

CASE ePMLState OF
	
// =========================================================
	// Turning axis reset off, passing it to axis instances
	ePMLState_IDLE:
	
				IF bResetStart THEN
					bResetStart 			:= FALSE;
					
					fbSeparateModule.bReset	:= FALSE;
					fbSeparateModule.M_Reset();
					
					fbMetalSorting.bReset 	:= FALSE;							
					fbMetalSorting.M_Reset();
					
					fbPlasticSorting.bReset := FALSE;							
					fbPlasticSorting.M_Reset();
					
					fbStateMachineAuto.StateComplete := FALSE;	
				END_IF
	
// =========================================================
	// Resetting variables for executing automatic mode, checking status of axes
	ePMLState_STARTING:
	
				IF NOT bStartingStart THEN
					bStartingStart 				:= TRUE;
					
					fbSeparateModule.bStarting 	:= TRUE;							
					fbSeparateModule.M_Starting();
					
					fbMetalSorting.bStarting 	:= TRUE;							
					fbMetalSorting.M_Starting();
					
					fbPlasticSorting.bStarting 	:= TRUE;							
					fbPlasticSorting.M_Starting();
				END_IF

				IF NOT fbSeparateModule.bStartingDone THEN
					fbSeparateModule.M_Starting();
				END_IF
				
				IF NOT fbMetalSorting.bStartingDone THEN
					fbMetalSorting.M_Starting();
				END_IF
				
				IF NOT fbPlasticSorting.bStartingDone THEN
					fbPlasticSorting.M_Starting();
				END_IF

				IF fbSeparateModule.bStartingDone AND fbMetalSorting.bStartingDone
				AND fbPlasticSorting.bStartingDone THEN
					fbStateMachineAuto.StateComplete := TRUE;
				END_IF

// =========================================================
	// Executing automatic mode
	ePMLState_EXECUTE:	

				IF bStartingStart THEN
					bStartingStart 				:= FALSE;
					
					fbSeparateModule.bStarting 	:= FALSE;							
					fbSeparateModule.M_Starting();
					
					fbMetalSorting.bStarting 	:= FALSE;							
					fbMetalSorting.M_Starting();
					
					fbPlasticSorting.bStarting 	:= FALSE;							
					fbPlasticSorting.M_Starting();
					
					fbStateMachineAuto.StateComplete := FALSE;
				END_IF
				
				fbSeparateModule.M_Automatic();
				fbMetalSorting.M_Automatic();
				fbPlasticSorting.M_Automatic();
				
				IF fbTriggerSeparated.Q THEN
					nBoxesOnTheWay := nBoxesOnTheWay + 1;
				END_IF
				
				IF fbTriggerSelectedM.Q THEN
					nBoxesOnTheWay := nBoxesOnTheWay - 1;
				END_IF
				
				IF fbTriggerSelectedP.Q THEN
					nBoxesOnTheWay := nBoxesOnTheWay - 1;
				END_IF
						
// =========================================================
	// Stopping axes
	ePMLState_ABORTING:

				IF NOT bHaltStart THEN
					bHaltStart 				:= TRUE;
					
					fbSeparateModule.bHalt 	:= TRUE;							
					fbSeparateModule.M_Stop();
					
					fbMetalSorting.bHalt 	:= TRUE;							
					fbMetalSorting.M_Stop();
					
					fbPlasticSorting.bHalt 	:= TRUE;							
					fbPlasticSorting.M_Stop();						
				END_IF

				IF NOT fbSeparateModule.bHaltDone THEN
					fbSeparateModule.M_Stop();
				END_IF
				
				IF NOT fbMetalSorting.bHaltDone THEN
					fbMetalSorting.M_Stop();
				END_IF
				
				IF NOT fbPlasticSorting.bHaltDone THEN
					fbPlasticSorting.M_Stop();
				END_IF

				IF fbSeparateModule.bHaltDone AND fbMetalSorting.bHaltDone
				AND fbPlasticSorting.bHaltDone THEN
					fbStateMachineAuto.StateComplete := TRUE;
				END_IF
	
// =========================================================
	// Turning off axis stop, passing it to axis instances
	ePMLState_ABORTED:

				IF fbStateMachineAuto.StateComplete THEN
					fbStateMachineAuto.StateComplete := FALSE;
				END_IF
				
				IF bHaltStart THEN
					bHaltStart 				:= FALSE;
					
					fbSeparateModule.bHalt 	:= FALSE;							
					fbSeparateModule.M_Stop();
					
					fbMetalSorting.bHalt 	:= FALSE;							
					fbMetalSorting.M_Stop();
					
					fbPlasticSorting.bHalt 	:= FALSE;							
					fbPlasticSorting.M_Stop();
				END_IF
	
// =========================================================
	ePMLState_CLEARING:

				fbStateMachineAuto.StateComplete := TRUE;
	
// =========================================================
	// Selecting boxes on conveyor belt to destination, then stopping axes
	ePMLState_STOPPING:	

				IF fbTriggerSeparated.Q THEN
					nBoxesOnTheWay := nBoxesOnTheWay + 1;
				END_IF
				
				IF fbTriggerSelectedM.Q THEN
					nBoxesOnTheWay := nBoxesOnTheWay - 1;
				END_IF
				
				IF fbTriggerSelectedP.Q THEN
					nBoxesOnTheWay := nBoxesOnTheWay - 1;
				END_IF
				
				IF nBoxesOnTheWay = 0 AND NOT bHaltStart THEN
					bHaltStart 				:= TRUE;
					
					fbSeparateModule.bHalt 	:= TRUE;							
					fbSeparateModule.M_Stop();
					
					fbMetalSorting.bHalt 	:= TRUE;							
					fbMetalSorting.M_Stop();
					
					fbPlasticSorting.bHalt 	:= TRUE;							
					fbPlasticSorting.M_Stop();			
				END_IF
				
				IF NOT fbSeparateModule.bHaltDone OR nBoxesOnTheWay <> 0 THEN
					fbSeparateModule.M_Automatic();
				END_IF
				
				IF NOT fbMetalSorting.bHaltDone OR nBoxesOnTheWay <> 0 THEN
					fbMetalSorting.M_Automatic();
				END_IF
				
				IF NOT fbPlasticSorting.bHaltDone OR nBoxesOnTheWay <> 0 THEN
					fbPlasticSorting.M_Automatic();
				END_IF

				IF fbSeparateModule.bHaltDone AND fbMetalSorting.bHaltDone
				AND fbPlasticSorting.bHaltDone AND nBoxesOnTheWay = 0 THEN
					fbStateMachineAuto.StateComplete := TRUE;
				END_IF
					
// =========================================================
	// Turning off axis stop, passing it to axis instances
	ePMLState_STOPPED:	

				IF fbStateMachineAuto.StateComplete THEN
					fbStateMachineAuto.StateComplete := FALSE;	
				END_IF
				
				IF bHaltStart THEN
					bHaltStart 				:= FALSE;
					
					fbSeparateModule.bHalt 	:= FALSE;							
					fbSeparateModule.M_Stop();
					
					fbMetalSorting.bHalt 	:= FALSE;							
					fbMetalSorting.M_Stop();
					
					fbPlasticSorting.bHalt 	:= FALSE;							
					fbPlasticSorting.M_Stop();
				END_IF

// =========================================================
	// Resetting cylinders and axes
	ePMLState_RESETTING:	

				IF NOT bResetStart THEN
					bResetStart 			:= TRUE;
					
					fbSeparateModule.bReset	:= TRUE;
					fbSeparateModule.M_Reset();
					
					fbMetalSorting.bReset 	:= TRUE;
					fbMetalSorting.M_Reset();
					
					fbPlasticSorting.bReset	:= TRUE;
					fbPlasticSorting.M_Reset();
				END_IF
				
				IF NOT fbSeparateModule.bResetDone THEN
					fbSeparateModule.M_Reset();
				END_IF
				
				IF NOT fbMetalSorting.bResetDone THEN
					fbMetalSorting.M_Reset();
				END_IF
				
				IF NOT fbPlasticSorting.bResetDone THEN
					fbPlasticSorting.M_Reset();
				END_IF
				
				IF fbSeparateModule.bResetDone AND fbMetalSorting.bResetDone AND fbPlasticSorting.bResetDone 
				AND fbSeparateModule.bClampAtBase AND fbSeparateModule.bBarrierAtBase
				AND fbMetalSorting.bAtBase AND fbPlasticSorting.bAtBase THEN
					nBoxesOnTheWay 						:= 0;
					fbStateMachineAuto.StateComplete 	:= TRUE;
				END_IF
END_CASE

// =========================================================
END_ACTION

END_PROGRAM
